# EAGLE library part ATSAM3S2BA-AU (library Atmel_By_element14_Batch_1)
Flash MCU
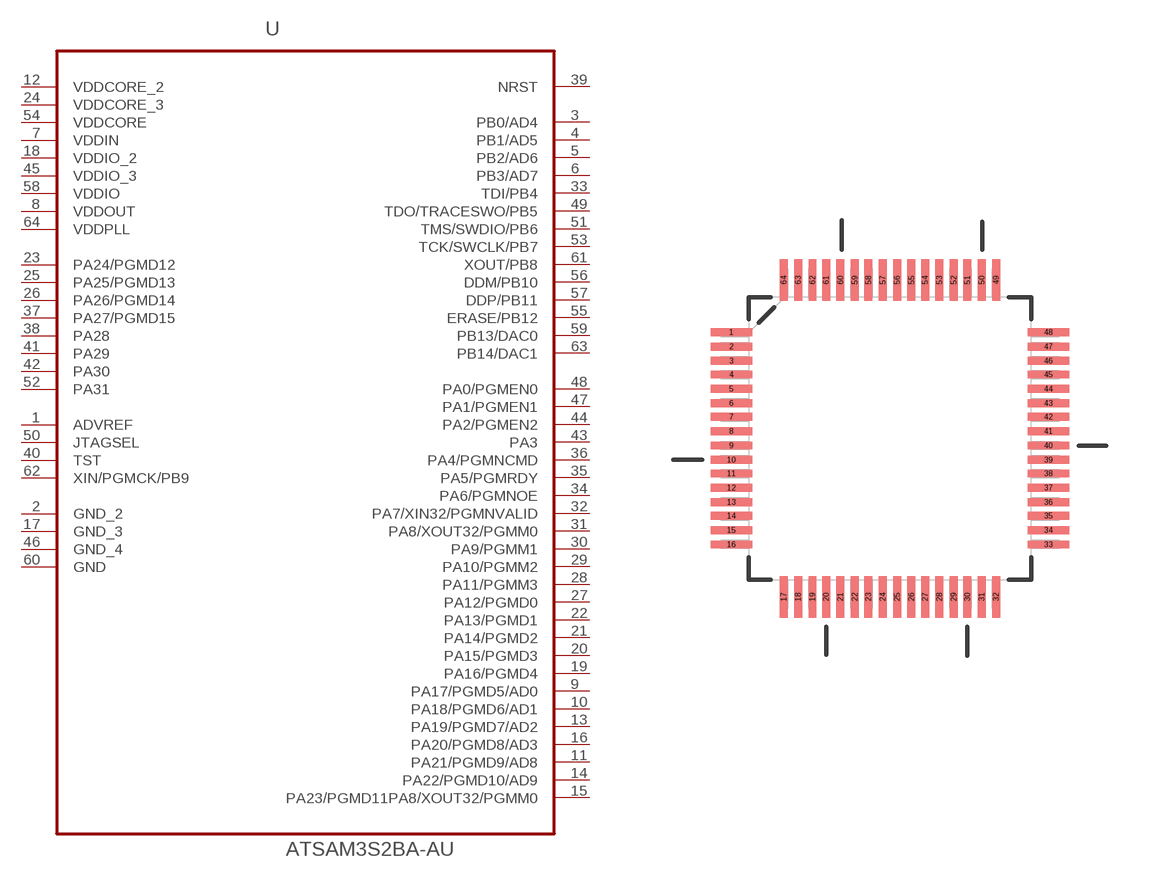
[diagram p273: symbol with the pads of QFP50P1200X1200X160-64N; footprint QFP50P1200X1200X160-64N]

Designator prefix U

## ATSAM3S2BA-AU (DESCRIPTION: Flash MCU; MPN: ATSAM3S2BA-AU; OC_FARNELL: 1841653; OC_NEWARK: 12T1311; PACKAGE: QFP-64; SUPPLIER: Atmel)  [QFP50P1200X1200X160-64N]
1  ADVREF  in
2  GND_2  pas
3  PB0/AD4
4  PB1/AD5
5  PB2/AD6
6  PB3/AD7
7  VDDIN  pwr
8  VDDOUT  pwr
9  PA17/PGMD5/AD0
10  PA18/PGMD6/AD1
11  PA21/PGMD9/AD8
12  VDDCORE_2  pwr
13  PA19/PGMD7/AD2
14  PA22/PGMD10/AD9
15  PA23/PGMD11PA8/XOUT32/PGMM0
16  PA20/PGMD8/AD3
17  GND_3  pas
18  VDDIO_2  pwr
19  PA16/PGMD4
20  PA15/PGMD3
21  PA14/PGMD2
22  PA13/PGMD1
23  PA24/PGMD12
24  VDDCORE_3  pwr
25  PA25/PGMD13
26  PA26/PGMD14
27  PA12/PGMD0
28  PA11/PGMM3
29  PA10/PGMM2
30  PA9/PGMM1
31  PA8/XOUT32/PGMM0
32  PA7/XIN32/PGMNVALID
33  TDI/PB4
34  PA6/PGMNOE
35  PA5/PGMRDY
36  PA4/PGMNCMD
37  PA27/PGMD15
38  PA28
39  NRST
40  TST  in
41  PA29
42  PA30
43  PA3
44  PA2/PGMEN2
45  VDDIO_3  pwr
46  GND_4  pas
47  PA1/PGMEN1
48  PA0/PGMEN0
49  TDO/TRACESWO/PB5
50  JTAGSEL  in
51  TMS/SWDIO/PB6
52  PA31
53  TCK/SWCLK/PB7
54  VDDCORE  pwr
55  ERASE/PB12
56  DDM/PB10
57  DDP/PB11
58  VDDIO  pwr
59  PB13/DAC0
60  GND  pas
61  XOUT/PB8  out
62  XIN/PGMCK/PB9  in
63  PB14/DAC1
64  VDDPLL  pwr

## Footprint QFP50P1200X1200X160-64N (pad centres in mm)
smd 1.473 x 0.279: 1 -5.613,3.759; 2 -5.613,3.251; 3 -5.613,2.743; 4 -5.613,2.261; 5 -5.613,1.753; 6 -5.613,1.245; 7 -5.613,0.762; 8 -5.613,0.254; 9 -5.613,-0.254; 10 -5.613,-0.762; 11 -5.613,-1.245; 12 -5.613,-1.753; 13 -5.613,-2.261; 14 -5.613,-2.743; 15 -5.613,-3.251; 16 -5.613,-3.759; 33 5.613,-3.759; 34 5.613,-3.251; 35 5.613,-2.743; 36 5.613,-2.261; 37 5.613,-1.753; 38 5.613,-1.245; 39 5.613,-0.762; 40 5.613,-0.254; 41 5.613,0.254; 42 5.613,0.762; 43 5.613,1.245; 44 5.613,1.753; 45 5.613,2.261; 46 5.613,2.743; 47 5.613,3.251; 48 5.613,3.759
smd 0.279 x 1.473: 17 -3.759,-5.613; 18 -3.251,-5.613; 19 -2.743,-5.613; 20 -2.261,-5.613; 21 -1.753,-5.613; 22 -1.245,-5.613; 23 -0.762,-5.613; 24 -0.254,-5.613; 25 0.254,-5.613; 26 0.762,-5.613; 27 1.245,-5.613; 28 1.753,-5.613; 29 2.261,-5.613; 30 2.743,-5.613; 31 3.251,-5.613; 32 3.759,-5.613; 49 3.759,5.613; 50 3.251,5.613; 51 2.743,5.613; 52 2.261,5.613; 53 1.753,5.613; 54 1.245,5.613; 55 0.762,5.613; 56 0.254,5.613; 57 -0.254,5.613; 58 -0.762,5.613; 59 -1.245,5.613; 60 -1.753,5.613; 61 -2.261,5.613; 62 -2.743,5.613; 63 -3.251,5.613; 64 -3.759,5.613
